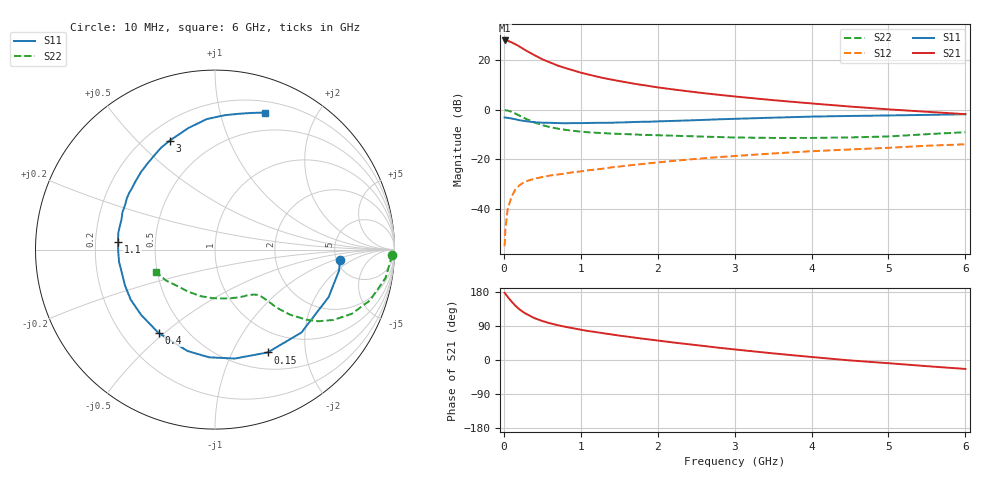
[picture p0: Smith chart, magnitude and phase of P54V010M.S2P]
! SIEMENS Small Signal Semiconductors
! BFP183
! Si NPN RF Bipolar Junction Transistor in SOT143
! VCE = 4 V  IC = 10 mA
! Common Emitter S-Parameters:  March  1996
# GHz  S  MA  R  50
!  f  S11  S21  S12  S22
! GHz  MAG  ANG  MAG  ANG  MAG  ANG  MAG  ANG
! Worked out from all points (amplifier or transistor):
!   36 points, 10 MHz to 6 GHz, reference 50 ohm
!   highest |S21| = 27.9 dB at 10 MHz (marker M1)
!   |S21| within 3 dB of that: start of sweep to 231.7 MHz
!   unconditionally stable (mu >= 1): 1.185 GHz to 5.605 GHz
!   at 250 MHz: K = 0.32, MSG = 27.0 dB, |S12| = -29.4 dB
!   at 1.4 GHz: K = 1.07, MAG = 16.1 dB, |S12| = -23.2 dB
!   at 6 GHz: K = 0.95, MSG = 6.1 dB, |S12| = -13.9 dB
!   lowest NFmin = 1.30 dB at 450 MHz
!   S11 on the Smith chart (normalised r, x): 10 MHz: 5.39, -1.19; 150 MHz: 0.71, -1.38; 400 MHz: 0.35, -0.48; 1.1 GHz: 0.30, +0.03; 3 GHz: 0.29, +0.63; 6 GHz: 0.31, +1.38
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0.01  0.6998 -4.6  24.82 177.2  0.0018 89.2  0.9859 -1.8
0.02  0.7012 -9.5  24.72 174.9  0.0039 80.1  0.9793 -3.9
0.05  0.6862 -22.7  24.46 166.5  0.01 83.0  0.9629 -9.5
0.1  0.6673 -43.8  22.76 154.3  0.0178 69.1  0.9082 -18.2
0.15  0.6438 -62.9  20.87 143.3  0.0248 61.9  0.8415 -25.2
0.2  0.6169 -79.7  18.9 134.1  0.0299 56.9  0.7675 -30.7
0.25  0.601 -93.2  16.85 126.7  0.0339 51.7  0.7013 -34.7
0.3  0.5855 -105.1  15.21 120.7  0.0368 48.6  0.6441 -37.4
0.4  0.5612 -124.0  12.5 110.4  0.0411 44.7  0.5543 -40.9
0.5  0.5493 -138.4  10.4 102.9  0.0442 42.2  0.4912 -42.7
0.6  0.5463 -149.3  8.967 97.0  0.0475 41.7  0.4482 -43.6
0.7  0.5398 -158.4  7.755 92.0  0.0497 41.5  0.4175 -44.1
0.8  0.5349 -166.0  6.92 87.5  0.0522 41.3  0.3948 -44.5
1.1  0.542 175.7  5.125 76.4  0.0606 42.4  0.3524 -46.2
1.5  0.5563 158.0  3.783 64.4  0.0719 43.2  0.3271 -50.1
1.8  0.5731 146.5  3.155 56.3  0.0809 43.5  0.3131 -54.3
2.2  0.5971 133.8  2.569 46.3  0.0933 42.1  0.3005 -61.2
3  0.6574 112.6  1.853 27.9  0.1173 38.2  0.277 -78.8
3.5  0.6936 102.3  1.561 17.5  0.1321 35.0  0.2712 -91.9
4.5  0.7504 86.0  1.161 -1.1  0.159 27.7  0.2776 -121.9
5.5  0.7891 74.8  0.911 -16.3  0.1888 21.1  0.3226 -147.7
6  0.8127 70.0  0.816 -23.6  0.202 16.8  0.3535 -159.2
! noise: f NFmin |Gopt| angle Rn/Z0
0.45  1.3  0.15  45  0.18
0.9  1.4  0.2  125  0.19
1.8  2.1  0.34  -170  0.14
